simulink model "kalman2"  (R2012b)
settings: Solver=ode45  StartTime=0.0  StopTime=50.0  RelTol=1e-3
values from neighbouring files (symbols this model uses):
  A1 = 0.02    [fuellstnd_1.m]    (also in fuellstnd_2.m; fuellstnd_21.m; fuellstnd_3.m; fuellstnd_31.m)
  A2 = A1    (= 0.02)    [fuellstnd_1.m]    (also in fuellstnd_2.m; fuellstnd_21.m; fuellstnd_3.m; fuellstnd_31.m)
  B1 = sys1.b    [kalman_11.m]    (also in kalman_12.m; kalman_13.m; kalman_2.m; kalman_3.m)
  B2 = sys2.b    [kalman_2.m]    (also in kalman_3.m)
  C1 = sys1.c    [kalman_11.m]    (also in kalman_12.m; kalman_13.m; kalman_2.m; kalman_3.m)
  C2 = sys2.c    [kalman_2.m]    (also in kalman_3.m; feder_masse_1.m = [0 0 1 0]; feder_masse_13.m = [0 0 1 0]; feder_masse_14.m = [0 0 1 0])
  dt = 0.01    [aktiv_tilger_1.m]    (also in aktiv_tilger_12.m; aktiv_tilger_2.m; beobachter_1.m; beobachter_2.m)
  Kest = kalman(P,1,0.01),    [LQG_1.m]    (also in ss_zwei_eing_1.m = kalman(sys2, Q, R))
  vnd = 1e-4    (= 0.0001)    [kalman_1.m]    (also in kalman_10.m; kalman_11.m; kalman_12.m; kalman_13.m = 0.01)
  vny = 1e-6    (= 1e-06)    [kalman_1.m]    (also in kalman_10.m; kalman_11.m = ', num2str(vny),' )']); kalman_12.m = ', num2str(vny),' )']); kalman_13.m = ', num2str(vny),' )']))
libraries: simulink x2, dspstat3 x1

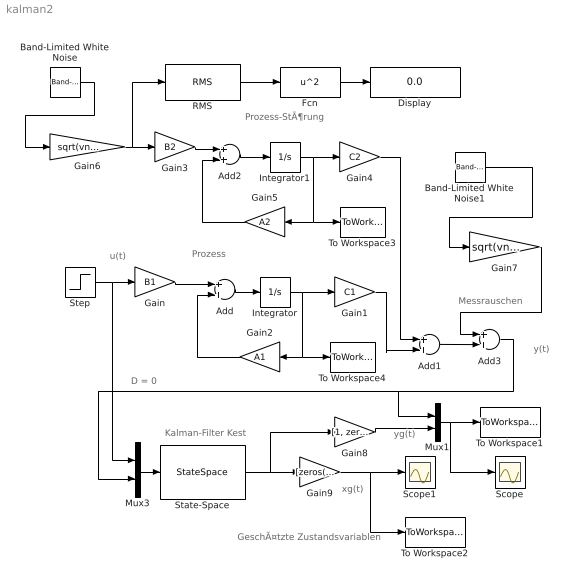
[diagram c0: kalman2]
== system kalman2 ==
  note: Prozess
  note: Prozess-StÃ¶rung
  note: Messrauschen
  note: xg(t)
  note: y(t)
  note: u(t)
  note: D = 0
  note: Kalman-Filter Kest
  note: yg(t)
  note: GeschÃ¤tzte Zustandsvariablen
  Add{,1..3} (4 alike) : Sum
  Band-Limited White Noise : simulink/Sources/Band-Limited White Noise  Cov=dt  Ts=dt  seed=[23341]
  Band-Limited White Noise1 : simulink/Sources/Band-Limited White Noise  Cov=dt  Ts=dt  seed=[23341]
  Display : Display
  Fcn : Fcn  Expr=u^2
  Gain : Gain  Gain=B1  Multiplication=Matrix(K*u)
  Gain1 : Gain  Gain=C1  Multiplication=Matrix(K*u)
  Gain2 : Gain  Gain=A1  Multiplication=Matrix(K*u)
  Gain3 : Gain  Gain=B2  Multiplication=Matrix(K*u)
  Gain4 : Gain  Gain=C2  Multiplication=Matrix(K*u)
  Gain5 : Gain  Gain=A2  Multiplication=Matrix(K*u)
  Gain6 : Gain  Gain=sqrt(vnd)
  Gain7 : Gain  Gain=sqrt(vny)
  Gain8 : Gain  Gain=[1, zeros(1,6)]  Multiplication=Matrix(K*u)
  Gain9 : Gain  Gain=[zeros(6,1),eye(6,6)]  Multiplication=Matrix(K*u)
  Integrator : Integrator
  Integrator1 : Integrator
  Mux1 : Mux  Inputs=2
  Mux3 : Mux  Inputs=2
  RMS : dspstat3/RMS  run=on  reset_popup=None  InputProcessing=Columns as channels (frame based)  directionMode=Each column  dimension=1  treatSBRowAsCol=on
  Scope : Scope
  Scope1 : Scope
  State-Space : StateSpace  A=Kest.a  B=Kest.b  C=Kest.c  D=Kest.d
  Step : Step  SampleTime=0
  To Workspace1 : ToWorkspace  VariableName=y1  SaveFormat=Structure With Time
  To Workspace2 : ToWorkspace  VariableName=y  SaveFormat=Structure With Time
  To Workspace3 : ToWorkspace  VariableName=y2  SaveFormat=Structure With Time
  To Workspace4 : ToWorkspace  VariableName=y3  SaveFormat=Structure With Time
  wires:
  Gain/1 -> Add/1
  Add/1 -> Integrator/1
  Integrator/1 -> To Workspace4/1, Gain2/1, Gain1/1
  Gain2/1 -> Add/2
  Gain6/1 -> RMS/1, Gain3/1
  Gain3/1 -> Add2/1
  Add2/1 -> Integrator1/1
  Integrator1/1 -> Gain4/1, To Workspace3/1, Gain5/1
  Gain5/1 -> Add2/2
  Band-Limited White Noise/1 -> Gain6/1
  Band-Limited White Noise1/1 -> Gain7/1
  Gain9/1 -> To Workspace2/1, Scope1/1
  Step/1 -> Mux3/1, Gain/1
  State-Space/1 -> Gain8/1, Gain9/1
  Add1/1 -> Add3/2
  Mux3/1 -> State-Space/1
  Gain7/1 -> Add3/1
  Mux1/1 -> Scope/1, To Workspace1/1
  Add3/1 -> Mux3/2, Mux1/1
  Gain8/1 -> Mux1/2
  Gain4/1 -> Add1/1
  Gain1/1 -> Add1/2
  RMS/1 -> Fcn/1
  Fcn/1 -> Display/1
